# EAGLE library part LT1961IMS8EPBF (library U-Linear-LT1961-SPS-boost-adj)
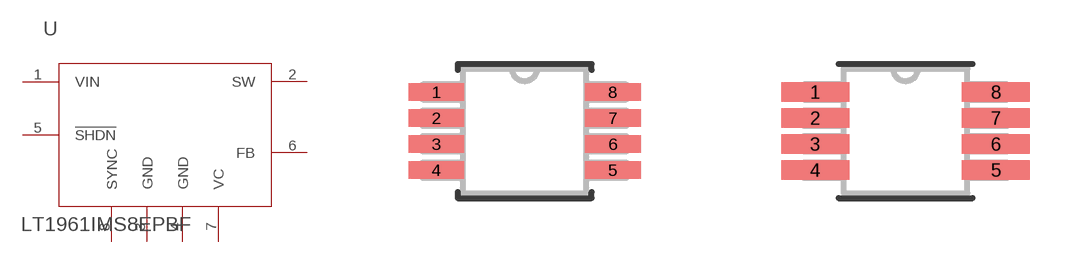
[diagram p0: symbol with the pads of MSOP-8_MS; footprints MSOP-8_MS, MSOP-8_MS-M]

Designator prefix U

## LT1961IMS8EPBF (MANUFACTURER_PART_NUMBER: LT1961; VALUE: LT1961; VENDOR: Linear Technology)  [MSOP-8_MS]
1  VIN  in
2  SW  pas
3  GND  pwr
4  GND  pwr
5  !SHDN  in
6  FB  out
7  VC  out
8  SYNC  pas

## LT1961IMS8EPBFMSOP-8_MS-M (MANUFACTURER_PART_NUMBER: LT1961IMS8E#PBF; VENDOR: Linear Technology)  [MSOP-8_MS-M]
Pads as for MSOP-8_MS

## LT1961IMS8EPBFMSOP-8_MS-L (MANUFACTURER_PART_NUMBER: LT1961IMS8E#PBF; VENDOR: Linear Technology)  [MSOP-8_MS-L]
Pads as for MSOP-8_MS

## Footprint MSOP-8_MS (pad centres in mm)
smd 1.397 x 0.432: 1 -2.21,0.975; 2 -2.21,0.325; 3 -2.21,-0.325; 4 -2.21,-0.975; 5 2.21,-0.975; 6 2.21,-0.325; 7 2.21,0.325; 8 2.21,0.975

## Footprint MSOP-8_MS-M (pad centres in mm)
smd 1.702 x 0.483: 1 -2.261,0.975; 2 -2.261,0.325; 3 -2.261,-0.325; 4 -2.261,-0.975; 5 2.261,-0.975; 6 2.261,-0.325; 7 2.261,0.325; 8 2.261,0.975

## Footprint MSOP-8_MS-L (pad centres in mm)
smd 1.092 x 0.381: 1 -2.159,0.975; 2 -2.159,0.325; 3 -2.159,-0.325; 4 -2.159,-0.975; 5 2.159,-0.975; 6 2.159,-0.325; 7 2.159,0.325; 8 2.159,0.975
